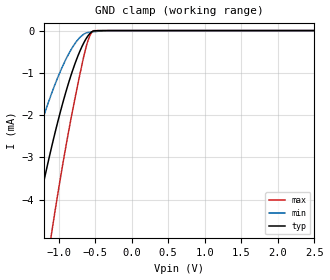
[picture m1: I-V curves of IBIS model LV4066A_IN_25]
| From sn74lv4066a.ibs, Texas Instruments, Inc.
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[Model]   LV4066A_IN_25
Model_type  Input
Vinl = 0.69
Vinh = 1.89
| variable   typ   min   max
C_comp   1.26pF   0.81pF   1.46pF
[Temperature Range]   40   100   -40
| Ambient temperature   25   85   -40
[Voltage range]   2.5   2.3   2.7
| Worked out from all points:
|   GND clamp passes 1 mA (typ) near -0.82 V on its own axis
[GND Clamp]
| LV4066A_IN_25
|   Voltage   I(typ)   I(min)   I(max)
-2.5V     -17.05mA   -11.36mA   -25.61mA
-1.66V    -7.706mA   -4.815mA   -12.15mA
-1.63V    -7.409mA   -4.61mA    -11.71mA
-1.335V   -4.669mA   -2.746mA   -7.68mA
-1.095V   -2.745mA   -1.481mA   -4.777mA
-975mV    -1.913mA   -958.1uA   -3.482mA
-855mV    -1.189mA   -528.2uA   -2.306mA
-750mV    -661.2uA   -245.3uA   -1.378mA
-645mV    -255.5uA   -74.6uA    -531.1uA
-575mV    -74.68uA   -38.44uA   -133.8uA
-515mV    -7.128uA   -26.16uA   -2.186uA
2.5V      10.21pA    144.7pA    7.51pA
